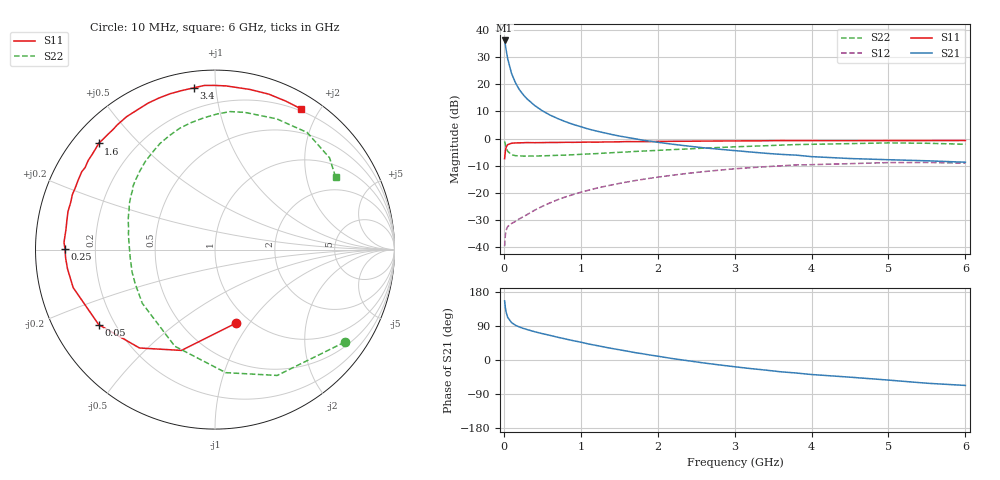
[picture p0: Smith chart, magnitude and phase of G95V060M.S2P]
! SIEMENS Small Signal Semiconductors
! BFG235
! Si NPN RF Bipolar Junction Transistor in SOT223
! VCE = 5 V  IC = 60 mA
! Common Emitter S-Parameters:  July  1994
# GHz  S  MA  R  50
!  f  S11  S21  S12  S22
! GHz  MAG  ANG  MAG  ANG  MAG  ANG  MAG  ANG
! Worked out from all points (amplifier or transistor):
!   40 points, 10 MHz to 6 GHz, reference 50 ohm
!   highest |S21| = 36.1 dB at 10 MHz (marker M1)
!   |S21| within 3 dB of that: start of sweep to 27.28 MHz
!   unconditionally stable (mu >= 1): 491.8 MHz to 1.363 GHz
!   at 200 MHz: K = 0.70, MSG = 23.9 dB, |S12| = -29.6 dB
!   at 1.5 GHz: K = 0.98, MSG = 8.7 dB, |S12| = -16.5 dB
!   at 6 GHz: K = 0.91, MSG = 0.2 dB, |S12| = -9.1 dB
!   S11 on the Smith chart (normalised r, x): 10 MHz: 0.86, -0.86; 50 MHz: 0.14, -0.29; 250 MHz: 0.09, +0.00; 1.6 GHz: 0.08, +0.39; 3.4 GHz: 0.08, +0.87; 6 GHz: 0.18, +1.77
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0.01  0.4259 -74.0  64.03 156.1  0.0104 68.2  0.8877 -35.5
0.02  0.5919 -108.4  52.58 138.4  0.0168 53.2  0.7821 -63.7
0.03  0.691 -127.5  42.88 126.2  0.0205 43.2  0.6882 -85.0
0.05  0.7712 -147.2  29.46 112.6  0.0239 33.3  0.5831 -112.6
0.1  0.8181 -165.0  15.85 98.7  0.0272 32.0  0.5036 -143.6
0.15  0.8288 -172.6  10.7 91.8  0.0297 35.8  0.4833 -157.0
0.2  0.8335 -176.7  8.018 87.3  0.033 39.2  0.4787 -164.6
0.25  0.8356 179.9  6.46 83.6  0.0361 43.2  0.4749 -169.6
0.3  0.8423 177.2  5.4 80.5  0.0395 46.6  0.4747 -173.6
0.4  0.8378 172.4  4.063 74.7  0.0478 50.6  0.4756 -179.1
0.5  0.8411 168.8  3.244 69.6  0.0563 52.9  0.4794 176.6
0.6  0.846 165.5  2.705 65.0  0.0652 53.8  0.4847 172.8
0.7  0.846 161.8  2.334 60.1  0.0747 54.4  0.4905 169.5
0.9  0.8511 156.4  1.824 51.1  0.0928 52.9  0.5029 163.7
1.1  0.8599 149.8  1.494 42.3  0.1117 50.8  0.5199 157.9
1.6  0.8775 137.6  1.051 23.5  0.1581 42.4  0.5649 144.6
2.2  0.8894 123.6  0.783 3.5  0.2116 30.0  0.6258 128.4
3.2  0.9051 101.9  0.566 -22.5  0.29 6.6  0.7191 100.9
3.4  0.909 97.5  0.535 -26.6  0.3023 1.6  0.7367 94.9
4.5  0.9132 77.7  0.428 -45.3  0.3446 -24.1  0.8055 64.8
5.5  0.9165 64.5  0.389 -61.3  0.3622 -46.5  0.8178 38.7
6  0.9188 58.7  0.366 -67.1  0.3511 -54.9  0.7839 31.0
